FUNCTION_BLOCK UpTyp
VAR_INPUT
END_VAR
VAR_OUTPUT
END_VAR

// NETWORK 1
// instruction list
LD      TRUE
R       deviceDown
S       deviceUp

// NETWORK 2
// instruction list
LD      T#2s
ST      timerUp.PT

// NETWORK 3
// instruction list
LD      TRUE
S       timerUp.IN
CAL     timerUp

END_FUNCTION_BLOCK
